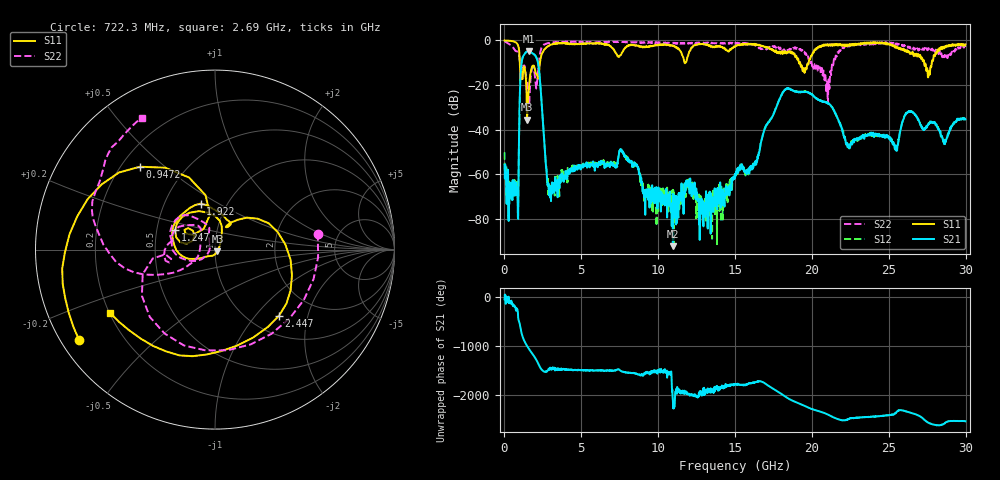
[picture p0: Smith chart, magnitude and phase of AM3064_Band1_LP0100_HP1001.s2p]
# Hz S DB R 50.0
!freq dBS11 angS11 dBS21 angS21 dBS12 angS12 dBS22 angS22
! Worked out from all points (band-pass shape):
!   1600 points, 10 MHz to 29.98 GHz, reference 50 ohm
!   highest |S21| = -4.83 dB at 1.584 GHz (marker M1); lowest = -92.2 dB at 10.96 GHz (marker M2)
!   |S21| within 3 dB of the highest: 1.174 GHz to 2.087 GHz (912.9 MHz wide, 56 % of centre)
!   lowest |S11| = -35.6 dB at 1.472 GHz (marker M3), VSWR 1.03, Z = 51.4 - j0.97 ohm
!   |S11| at or under -10 dB: 1.002 GHz to 2.308 GHz (1.306 GHz wide, 78.9 % of centre); 19.23 GHz to 19.79 GHz (557.8 MHz wide, 2.86 % of centre); 27.3 GHz to 27.8 GHz (495.8 MHz wide, 1.8 % of centre)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
!   |S22| runs from -30.3 to -0.4 dB; largest |S21 - S12| = 0.0086
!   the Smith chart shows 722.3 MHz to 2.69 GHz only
!   S11 on the Smith chart (normalised r, x): 722.3 MHz: 0.05, -0.30; 947.2 MHz: 0.27, +0.41; 1.247 GHz: 0.62, +0.14; 1.922 GHz: 0.75, +0.42; 2.447 GHz: 1.34, -1.34; 2.69 GHz: 0.20, -0.27
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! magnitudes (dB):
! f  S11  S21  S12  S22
! 10 MHz  0.0  -55.8  -50.2  -0.4
! 722.3 MHz  -0.8  -63.5  -66.8  -4.7
! 947.2 MHz  -4.1  -43.7  -43.7  -6.3
! 1.247 GHz  -12.1  -6.7  -6.7  -11.4
! 1.472 GHz  -35.6  -5.0  -4.9  -19.3
! 1.584 GHz  -21.2  -4.8  -4.9  -30.3
! 1.922 GHz  -11.4  -6.3  -6.2  -13.2
! 2.447 GHz  -5.8  -30.8  -30.7  -2.8
! 2.69 GHz  -3.3  -54.5  -55.3  -1.5
! 3.046 GHz  -1.8  -66.3  -65.1  -1.0
! 5.015 GHz  -1.4  -56.4  -56.5  -0.7
! 7.639 GHz  -5.5  -49.9  -49.9  -0.7
! 10 GHz  -2.0  -69.5  -68.3  -0.9
! 10.96 GHz  -2.3  -92.2  -67.0  -1.1
! 15 GHz  -2.7  -61.3  -59.7  -1.5
! 18.23 GHz  -5.7  -22.2  -22.1  -4.6
! 19.99 GHz  -6.9  -24.2  -24.1  -10.9
! 21.02 GHz  -1.8  -28.0  -28.1  -25.9
! 22.35 GHz  -1.9  -47.1  -46.8  -2.5
! 25 GHz  -1.3  -43.8  -43.7  -1.1
! 27.58 GHz  -14.7  -37.4  -37.1  -3.5
! 29.98 GHz  -1.8  -35.4  -35.0  -2.9
